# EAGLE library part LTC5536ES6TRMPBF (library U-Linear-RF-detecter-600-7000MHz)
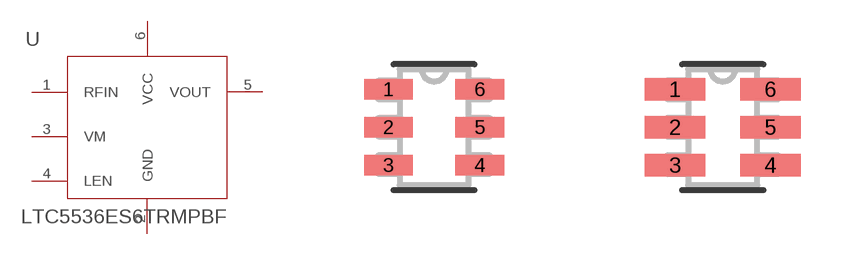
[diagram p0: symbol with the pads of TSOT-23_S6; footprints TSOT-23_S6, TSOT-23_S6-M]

Designator prefix U

## LTC5536ES6TRMPBF (MFR: Linear Technology; MPN: LTC5536; VALUE: LTC5536)  [TSOT-23_S6]
1  RFIN  in
2  GND  pwr
3  VM  in
4  LEN  in
5  VOUT  out
6  VCC  pwr

## LTC5536ES6TRMPBFTSOT-23_S6-M (MANUFACTURER_PART_NUMBER: LTC5536ES6#TRMPBF; VENDOR: Linear Technology)  [TSOT-23_S6-M]
Pads as for TSOT-23_S6

## LTC5536ES6TRMPBFTSOT-23_S6-L (MANUFACTURER_PART_NUMBER: LTC5536ES6#TRMPBF; VENDOR: Linear Technology)  [TSOT-23_S6-L]
Pads as for TSOT-23_S6

## Footprint TSOT-23_S6 (pad centres in mm)
smd 1.219 x 0.508: 1 -1.143,0.95; 2 -1.143,0; 3 -1.143,-0.95; 4 1.143,-0.95; 5 1.143,0; 6 1.143,0.95

## Footprint TSOT-23_S6-M (pad centres in mm)
smd 1.524 x 0.559: 1 -1.194,0.95; 2 -1.194,0; 3 -1.194,-0.95; 4 1.194,-0.95; 5 1.194,0; 6 1.194,0.95

## Footprint TSOT-23_S6-L (pad centres in mm)
smd 0.914 x 0.457: 1 -1.092,0.95; 2 -1.092,0; 3 -1.092,-0.95; 4 1.092,-0.95; 5 1.092,0; 6 1.092,0.95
